(* Logix 5000 AddOnInstructionDefinition export AMCI_SD4840E2_Resume; software revision 20.03 *)

ADD_ON_INSTRUCTION AMCI_SD4840E2_Resume   (* revision 1.0, vendor AMCI *)
VAR_IN_OUT
   AMCI_SD4840E2_output_data : _000A:SD4840E2_4342D302:O:0; {required}
END_VAR
VAR
   command_data_block : INT[10];
        [0]   // Command Bits MSW
        [1]   // Command Bits LSW
        [2]   // Upper Target Position
        [3]   // Lower Target Position
        [4]   // Upper Programmed Speed
        [5]   // Lower Programmed Speed
END_VAR

ROUTINE Logic   (* ladder *)
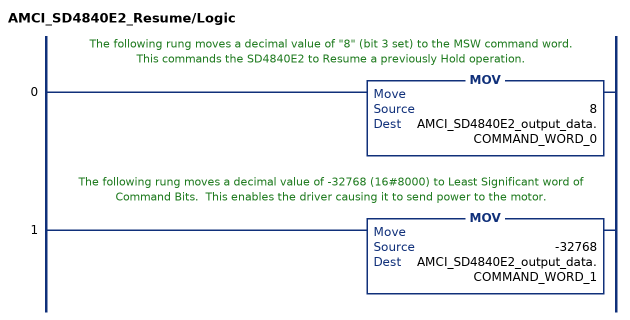
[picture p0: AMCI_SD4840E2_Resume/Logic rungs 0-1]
   // The following rung moves a decimal value of "8" (bit 3 set) to the MSW command word.  This commands the SD4840E2 to Resume a previously Hold operation.
   0: MOV(8,AMCI_SD4840E2_output_data.COMMAND_WORD_0);
   // The following rung moves a decimal value of -32768 (16#8000) to Least Significant word of Command Bits.  This enables the driver causing it to send power to the motor.
   1: MOV(-32768,AMCI_SD4840E2_output_data.COMMAND_WORD_1);
END_ROUTINE
END_ADD_ON_INSTRUCTION
